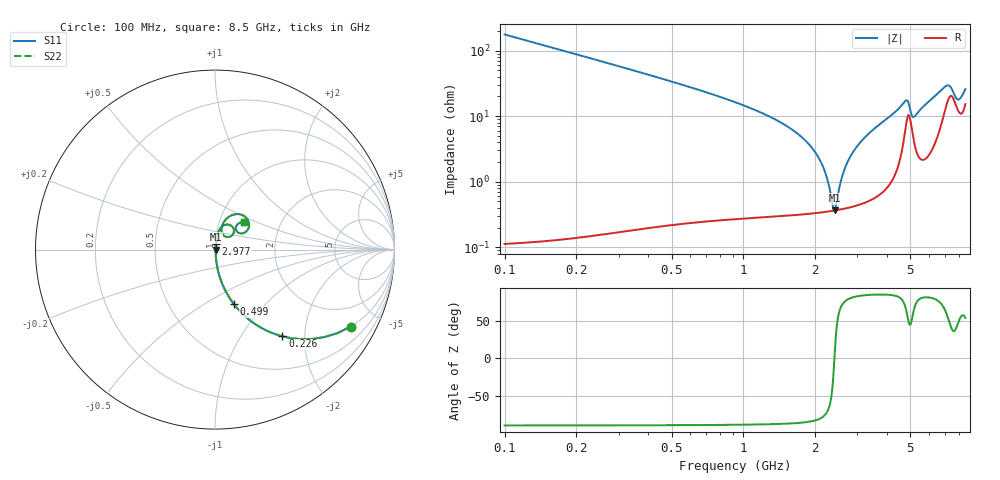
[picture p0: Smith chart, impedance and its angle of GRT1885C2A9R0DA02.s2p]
!Murata Part Number: GRT1885C2A9R0DA02
!These Parameters are Measured in Series Mode Connection
!Data Generated on Jun 19, 2026
!  o--ll--o
!Port1  Port2
!  o------o
!Operation Temp=25[degC], DC Bias Voltage=0[V]
!Freq. Start=100[MHz] Stop=9[GHz] 401[Steps]
# Hz S RI R 50
!Freq.(Hz) S11(Real) S11(Imag) S21(Real) S21(Imag) S12(Real) S12(Imag) S22(Real) S22(Imag)
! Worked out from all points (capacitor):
!   401 points, 100 MHz to 8.5 GHz, reference 50 ohm
!   read as one part in series: C = 9.01 pF near 142 MHz
!   lowest |Z| = 366 mohm at 2.41 GHz (marker M1)
!   series resonance near 2.405 GHz, so ESL is about 490 pH
!   S11 on the Smith chart (normalised r, x): 100 MHz: 1.00, -3.53; 226 MHz: 1.00, -1.55; 499 MHz: 1.00, -0.68; 2.977 GHz: 1.01, +0.07; 8.5 GHz: 1.31, +0.42
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1e8  0.7569 -0.4287  0.2431 0.4287  0.2431 0.4287  0.7569 -0.4287
2.26e8  0.3755 -0.4833  0.6245 0.4833  0.6245 0.4833  0.3755 -0.4833
3.31e8  0.216 -0.4098  0.784 0.4098  0.784 0.4098  0.216 -0.4098
4.99e8  0.1045 -0.3027  0.8955 0.3027  0.8955 0.3027  0.1045 -0.3027
8.98e8  0.0304 -0.1641  0.9696 0.1641  0.9696 0.1641  0.0304 -0.1641
1.507e9  0.00812 -0.0712  0.9919 0.0712  0.9919 0.0712  0.00812 -0.0712
1.843e9  0.00481 -0.0399  0.9952 0.0399  0.9952 0.0399  0.00481 -0.0399
2.074e9  0.00385 -0.0222  0.9961 0.0222  0.9961 0.0222  0.00385 -0.0222
2.221e9  0.00361 -0.0119  0.9964 0.0119  0.9964 0.0119  0.00361 -0.0119
2.368e9  0.0036 -0.00231  0.9964 0.00231  0.9964 0.00231  0.0036 -0.00231
2.41e9  0.00363 0.000345  0.9964 -0.000345  0.9964 -0.000345  0.00363 0.000345
2.641e9  0.00407 0.0143  0.9959 -0.0143  0.9959 -0.0143  0.00407 0.0143
2.914e9  0.00511 0.0299  0.9949 -0.0299  0.9949 -0.0299  0.00511 0.0299
2.977e9  0.00543 0.0333  0.9946 -0.0333  0.9946 -0.0333  0.00543 0.0333
3.46e9  0.00891 0.0594  0.9911 -0.0594  0.9911 -0.0594  0.00891 0.0594
4.3e9  0.0246 0.1095  0.9754 -0.1095  0.9754 -0.1095  0.0246 0.1095
4.804e9  0.0901 0.1331  0.9099 -0.1331  0.9099 -0.1331  0.0901 0.1331
5.14e9  0.0514 0.0766  0.9486 -0.0766  0.9486 -0.0766  0.0514 0.0766
5.707e9  0.04 0.134  0.96 -0.134  0.96 -0.134  0.04 0.134
7.114e9  0.1731 0.1783  0.8269 -0.1783  0.8269 -0.1783  0.1731 0.1783
7.891e9  0.1231 0.0999  0.8769 -0.0999  0.8769 -0.0999  0.1231 0.0999
8.5e9  0.1603 0.1523  0.8397 -0.1523  0.8397 -0.1523  0.1603 0.1523
